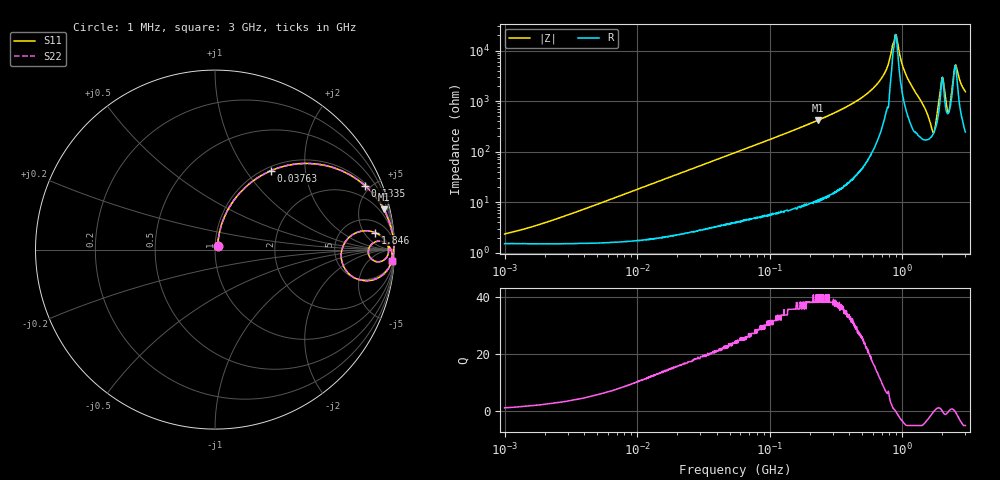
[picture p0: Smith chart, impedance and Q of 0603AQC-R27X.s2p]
!s-Parameter Generated by FASTRON Sdn. Bhd.
!FASTRON P/N : 0603AQC-R27X
!Keysight Technologies: E4991B_MY54100416_A.01.15
!Date: Thu Jun 25 14:07:08 2026
!Version  :Rev00  Thu Jun 25 14:07:08 2026
!Data & Calibration Information:
!Freq  S11  S21  S12  S22
!PortZ  Port1:50+j0  Port2:50+j0
!When reading reference impedance value at option line is always used.
! Remarks : This data is being provided solely for informational purposes.
# Hz S dB R 50
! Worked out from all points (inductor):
!   1601 points, 1 MHz to 3 GHz, reference 50 ohm
!   read as one part in series: L = 286 nH near 2.511 MHz
!   highest Q = 40.8 at 231.4 MHz (marker M1), where L = 287 nH
!   self-resonance near 893.7 MHz
!   S11 on the Smith chart (normalised r, x): 1 MHz: 1.03, +0.04; 37.63 MHz: 1.06, +1.32; 133.5 MHz: 1.14, +4.65; 1.846 GHz: 9, +9; 3 GHz: 6, -30
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1000000  -32.70 49.1  -0.13 -1.0  -0.13 -1.0  -32.70 49.1
3804036  -23.30 73.5  -0.15 -3.8  -0.15 -3.8  -23.30 73.5
1.447069e7  -12.20 71.5  -0.43 -14.1  -0.43 -14.1  -12.20 71.5
3.763315e7  -5.38 54.7  -1.75 -32.5  -1.75 -32.5  -5.38 54.7
5.504702e7  -3.38 45.0  -3.00 -42.6  -3.00 -42.6  -3.38 45.0
1.334721e8  -0.83 23.0  -8.15 -65.3  -8.15 -65.3  -0.83 23.0
2.083556e8  -0.36 14.9  -11.80 -73.6  -11.80 -73.6  -0.36 14.9
2.314421e8  -0.29 13.4  -12.70 -75.2  -12.70 -75.2  -0.29 13.4
5.445776e8  -0.05 4.0  -23.00 -83.3  -23.00 -83.3  -0.05 4.0
6.958997e8  -0.04 2.0  -29.00 -82.5  -29.00 -82.5  -0.04 2.0
7.925923e8  -0.02 1.0  -35.30 -80.2  -35.30 -80.2  -0.02 1.0
8.982141e8  -0.04 -0.0  -46.30 9.5  -46.30 9.5  -0.04 -0.0
1.064802e9  -0.06 -1.6  -30.60 76.6  -30.60 76.6  -0.06 -1.6
1.474099e9  -0.33 -7.2  -17.80 69.5  -17.80 69.5  -0.33 -7.2
1.662201e9  -1.87 -11.7  -11.50 37.9  -11.50 37.9  -1.87 -11.7
1.747494e9  -2.90 2.0  -10.90 -5.0  -10.90 -5.0  -2.90 2.0
1.846379e9  -0.96 6.1  -16.80 -41.0  -16.80 -41.0  -0.96 6.1
2.01032e9  -0.29 0.0  -29.70 -0.5  -29.70 -0.5  -0.29 0.0
2.177892e9  -0.93 -4.2  -18.20 32.4  -18.20 32.4  -0.93 -4.2
2.255531e9  -1.28 1.2  -17.20 -7.7  -17.20 -7.7  -1.28 1.2
2.543347e9  -0.15 -0.5  -34.30 26.9  -34.30 26.9  -0.15 -0.5
3e9  -0.11 -3.6  -23.80 77.2  -23.80 77.2  -0.11 -3.6
